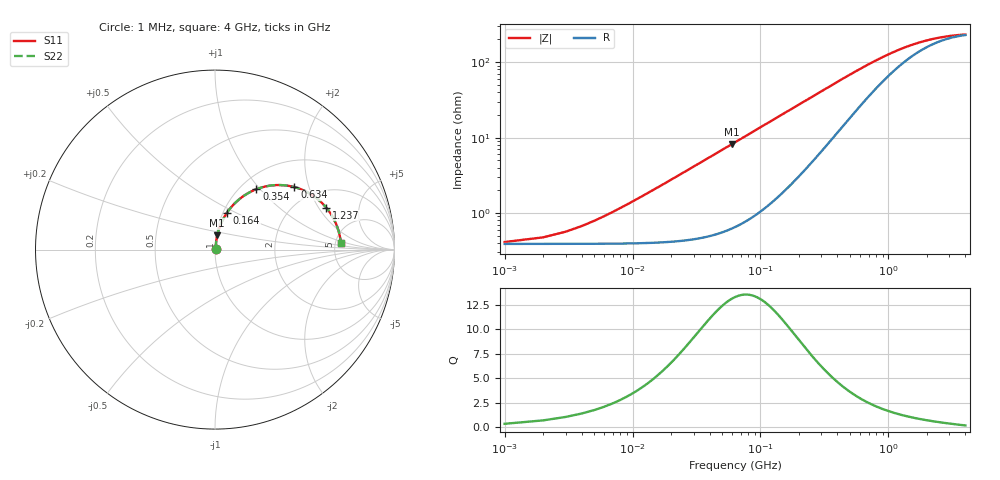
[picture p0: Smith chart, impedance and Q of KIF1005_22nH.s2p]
!version-2
!date-12.2020
!Series
# MHz S RI R 50
!Freq ReS11 ImS11 ReS21 ImS21 ReS12 ImS12 ReS22 ImS22
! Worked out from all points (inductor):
!   4000 points, 1 MHz to 4 GHz, reference 50 ohm
!   read as one part in series: L = 21.7 nH near 21 MHz
!   highest Q = 13.1 at 60 MHz (marker M1), where L = 21.7 nH
!   S11 on the Smith chart (normalised r, x): 1 MHz: 1.01, +0.00; 164 MHz: 1.04, +0.45; 354 MHz: 1.18, +0.96; 634 MHz: 1.58, +1.61; 1.237 GHz: 2.82, +2.35; 4 GHz: 5.58, +0.84
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1  0.00388 0.00136  0.9961 -0.00136  0.9961 -0.00136  0.00388 0.00136
11  0.00418 0.0149  0.9958 -0.0149  0.9958 -0.0149  0.00418 0.0149
24  0.00531 0.0325  0.9947 -0.0325  0.9947 -0.0325  0.00531 0.0325
30  0.00612 0.0405  0.9939 -0.0405  0.9939 -0.0405  0.00612 0.0405
43  0.00846 0.0579  0.9915 -0.0579  0.9915 -0.0579  0.00846 0.0579
60  0.0128 0.0804  0.9872 -0.0804  0.9872 -0.0804  0.0128 0.0804
79  0.0192 0.105  0.9808 -0.105  0.9808 -0.105  0.0192 0.105
103  0.0295 0.135  0.9705 -0.135  0.9705 -0.135  0.0295 0.135
131  0.0446 0.1683  0.9554 -0.1683  0.9554 -0.1683  0.0446 0.1683
164  0.0661 0.2046  0.9339 -0.2046  0.9339 -0.2046  0.0661 0.2046
248  0.1339 0.2796  0.8661 -0.2796  0.8661 -0.2796  0.1339 0.2796
354  0.2311 0.3367  0.7689 -0.3367  0.7689 -0.3367  0.2311 0.3367
478  0.3376 0.3593  0.6624 -0.3593  0.6624 -0.3593  0.3376 0.3593
634  0.4424 0.3482  0.5576 -0.3482  0.5576 -0.3482  0.4424 0.3482
668  0.4607 0.3427  0.5393 -0.3427  0.5393 -0.3427  0.4607 0.3427
917  0.5568 0.2934  0.4432 -0.2934  0.4432 -0.2934  0.5568 0.2934
1237  0.6199 0.2338  0.3801 -0.2338  0.3801 -0.2338  0.6199 0.2338
1334  0.6319 0.2185  0.3681 -0.2185  0.3681 -0.2185  0.6319 0.2185
2001  0.6751 0.1418  0.3249 -0.1418  0.3249 -0.1418  0.6751 0.1418
2667  0.6908 0.0951  0.3092 -0.0951  0.3092 -0.0951  0.6908 0.0951
3334  0.6978 0.0627  0.3022 -0.0627  0.3022 -0.0627  0.6978 0.0627
4000  0.7011 0.0382  0.2989 -0.0382  0.2989 -0.0382  0.7011 0.0382
